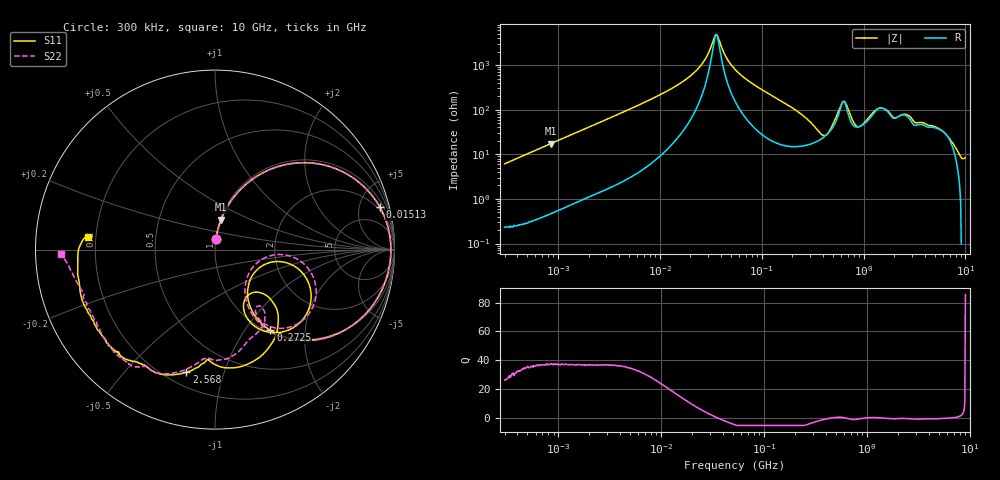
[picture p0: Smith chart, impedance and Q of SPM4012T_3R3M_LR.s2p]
! S-Parameter Data Generated by TDK Corporation
! Copyright(C) 2019 TDK Corporation.
! All Rights Reserved.
! TDK P/N: SPM4012T-3R3M-LR (Inductor)
! Property: L=3.3uH at 100kHz
! Size(LxWxT): 4.4x4.1x1.2mm
! Model Type: s2p (Touchstone File Format Version 1.0)
! Frequency: DC=Yes Start=0.3MHz Stop=10000MHz 802points Log-sweep
! Model Generated on Sep. 23, 2019
! Port Assignments:
!  1 ---@@@--- 2
! Applicable Conditions:
!  Temperature = 25 degC
!  DC Bias Current = 0 A
!  Small Signal Operation
! Terms and conditions regarding TDK Simulation Models
! (1)This simulation model is being provided solely for informational purposes. Please refer to the specifications of the products in terms of detailed characteristics of such products.
! (2)In no event shall TDK Corporation of any of its subsidiaries be liable for any loss or damage arising, directly or indirectly,
!  From any information contained in this simulation model, including, but not limited to loss or damages arising from any inaccuracies, omissions or errors in connection with such information.
! (3)Any and all copyrights on this simulation model are owned by TDK Corporation.
!  Duplication or redistribution of this simulation model without prior written permission from TDK Corporation is prohibited.
! (4)This simulation model is subject to any modification or change without any prior notice.
! (5)Neither TDK Corporation nor any of its subsidiaries shall make any warranty, express or implied,
!  Including but not limited to the correctness, implied warranties of merchantability and fitness for a particular purpose with respect to this simulation models.
! (6)The use of this simulation model shall be deemed to have consented to the terms and conditions hereof.
# Hz S MA R 50
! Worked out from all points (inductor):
!   801 points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, 300 kHz to 10 GHz, reference 50 ohm
!   read as one part in series: L = 3.24 uH near 318.3 kHz
!   highest Q = 37.4 at 857.3 kHz (marker M1), where L = 3.24 uH
!   self-resonance near 35.9 MHz
!   S11 on the Smith chart (normalised r, x): 300 kHz: 1.00, +0.12; 15.13 MHz: 1.59, +7.51; 272.5 MHz: 1.03, -1.32; 2.568 GHz: 0.28, -0.75; 10 GHz: 0.17, +0.05
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300000  0.05988 84.3  0.9958 -3.5  0.996 -3.5  0.05957 84.2
857268  0.1706 78.6  0.9807 -9.9  0.9809 -9.9  0.1705 78.6
1713600  0.3242 69.5  0.9372 -19.0  0.9373 -19.0  0.324 69.5
9671944  0.8855 25.1  0.4298 -62.6  0.4299 -62.6  0.8854 25.1
1.512819e7  0.9483 14.5  0.2613 -71.7  0.2614 -71.7  0.9482 14.5
2.53611e7  0.9769 4.6  0.099 -74.7  0.09906 -74.7  0.9768 4.6
3.555278e7  0.9799 -1.2  0.02029 -8.7  0.02028 -8.7  0.9798 -1.2
5.477226e7  0.9699 -8.9  0.1204 70.0  0.1205 70.0  0.9698 -8.9
1.585658e8  0.8092 -36.4  0.5109 47.5  0.511 47.5  0.8085 -36.7
2.725454e8  0.545 -55.6  0.7303 21.6  0.7305 21.6  0.5417 -56.4
3.126428e8  0.4528 -58.6  0.7675 13.5  0.7677 13.5  0.4476 -59.7
4.448526e8  0.2535 -33.6  0.7667 -11.7  0.767 -11.7  0.23 -33.2
5.344909e8  0.3865 -10.3  0.6342 -27.9  0.6344 -27.9  0.3639 -4.3
6.242396e8  0.6013 -27.1  0.393 -24.0  0.3931 -24.0  0.5979 -20.0
7.152593e8  0.5757 -53.5  0.4997 -0.5  0.4997 -0.5  0.6013 -45.8
8.643532e8  0.3652 -64.1  0.6598 -16.8  0.66 -16.8  0.43 -57.6
1.117505e9  0.3571 -42.9  0.5805 -39.8  0.5807 -39.8  0.4277 -51.0
1.387199e9  0.5607 -51.6  0.4166 -45.5  0.4167 -45.5  0.5201 -63.2
1.767019e9  0.6643 -83.2  0.4015 -38.5  0.4016 -38.6  0.5946 -79.2
2.568366e9  0.7013 -103.2  0.3375 -56.6  0.3375 -56.6  0.6932 -104.4
6.091595e9  0.7907 -142.7  0.2699 -90.0  0.2703 -90.1  0.7856 -144.5
1e10  0.71 174.5  0.1666 -128.0  0.1668 -128.2  0.8592 -178.2
